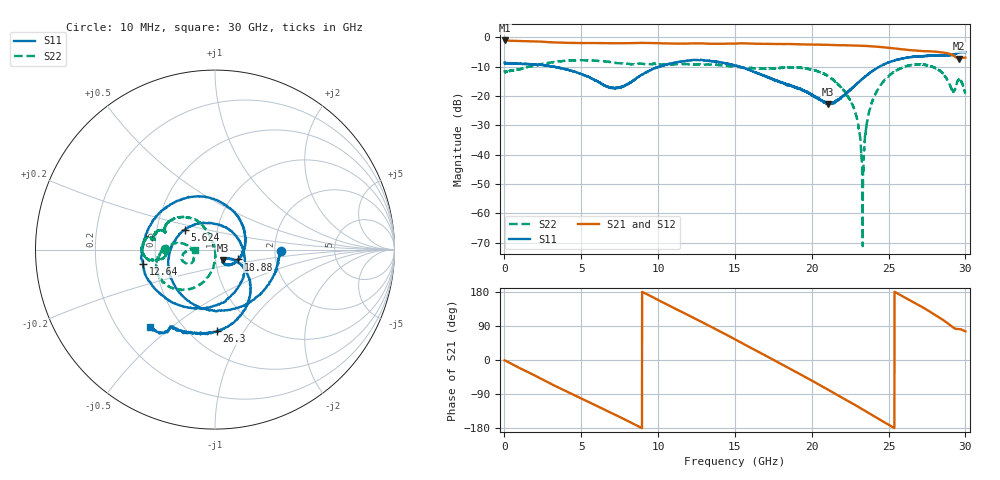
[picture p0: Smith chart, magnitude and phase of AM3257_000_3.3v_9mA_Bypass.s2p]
!Keysight Technologies,N5245B,MY58422270,A.16.20.02
!Date: Thursday, June 19, 2025 01:45:19
!Correction: S11(C  2-Port  )
!S21(C  2-Port  )
!S12(C  2-Port  )
!S22(C  2-Port  )
!S2P File: Measurements: S11, S21, S12, S22:
# Hz S  dB  R 50
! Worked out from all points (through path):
!   3201 points, 10 MHz to 30 GHz, reference 50 ohm
!   highest |S21| = -1.06 dB at 10 MHz (marker M1); lowest = -7.2 dB at 29.6 GHz (marker M2)
!   group delay of S21, straight-line fit = 59.7 ps
!   lowest |S11| = -22.7 dB at 21.06 GHz (marker M3), VSWR 1.16, Z = 54.3 - j6.31 ohm
!   |S11| at or under -10 dB: 3.191 GHz to 3.243 GHz (51.94 MHz wide, 1.61 % of centre); 3.243 GHz to 10.06 GHz (6.821 GHz wide, 103 % of centre); 15.31 GHz to 24.4 GHz (9.095 GHz wide, 45.8 % of centre)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
!   |S22| runs from -71.2 to -7.7 dB; largest |S21 - S12| = 0.026
!   S11 on the Smith chart (normalised r, x): 10 MHz: 2.17, -0.05; 5.624 GHz: 0.70, +0.16; 12.64 GHz: 0.42, -0.08; 18.88 GHz: 1.29, -0.15; 26.3 GHz: 0.67, -0.77; 30 GHz: 0.33, -0.42
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1e7  -8.63 -1.6  -1.06 -1.1  -1.22 -0.0  -11.14 179.4
2.277994e9  -9.36 -90.3  -1.42 -47.6  -1.54 -48.2  -9.31 -170.1
5.014581e9  -12.57 171.5  -1.95 -101.7  -1.97 -101.9  -7.79 178.7
5.623753e9  -13.96 147.5  -1.92 -113.4  -1.99 -113.5  -7.91 175.7
7.441897e9  -17.18 36.8  -2.02 -149.1  -2.02 -149.3  -8.84 169.3
1.000979e10  -10.09 -90.7  -1.99 158.2  -2.00 158.0  -9.28 170.1
1.264329e10  -7.75 -168.9  -2.06 104.3  -2.11 104.3  -9.26 165.1
1.5005e10  -9.58 120.8  -2.15 54.7  -2.17 54.7  -10.02 159.9
1.698247e10  -13.17 50.8  -2.22 11.8  -2.23 11.8  -10.63 160.9
1.888496e10  -17.00 -23.0  -2.30 -30.0  -2.47 -29.5  -10.29 153.6
2.000958e10  -19.44 -54.7  -2.44 -54.4  -2.44 -54.4  -11.01 141.7
2.105923e10  -22.74 -52.5  -2.56 -78.2  -2.51 -78.6  -13.20 127.4
2.268057e10  -17.12 -28.9  -2.79 -115.4  -2.78 -115.5  -23.29 110.9
2.301795e10  -15.41 -29.8  -2.83 -123.3  -2.83 -123.5  -29.15 106.8
2.330848e10  -14.19 -33.4  -2.88 -130.3  -2.89 -130.4  -62.00 -176.6
2.383331e10  -11.95 -41.2  -3.03 -142.9  -3.02 -143.1  -23.40 -90.7
2.500479e10  -8.57 -63.7  -3.56 -171.2  -3.54 -171.2  -13.19 -114.4
2.629811e10  -6.87 -88.5  -4.31 159.4  -4.32 159.3  -9.60 -141.6
2.819123e10  -6.10 -114.6  -4.97 114.9  -5.11 115.1  -10.84 179.2
2.919402e10  -5.96 -119.9  -6.13 86.1  -6.08 85.9  -18.37 -171.7
2.959701e10  -5.01 -123.7  -7.25 81.6  -7.35 82.0  -14.20 -161.8
3e10  -4.99 -130.0  -6.90 75.6  -6.88 74.3  -18.93 179.7
